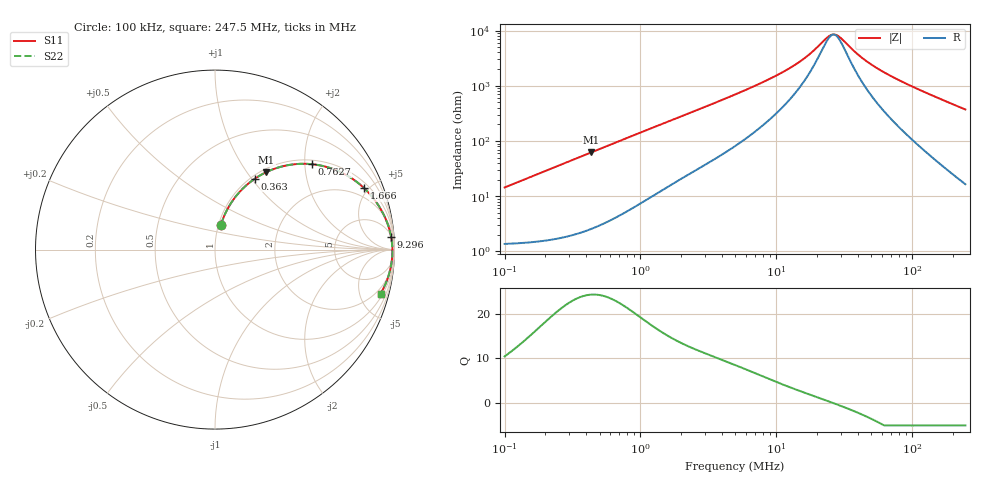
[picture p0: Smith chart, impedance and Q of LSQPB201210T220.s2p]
! LSQPB201210T220  S-PARAMETER MODEL  ( General Type )
! Model Generated by TAIYO YUDEN Corporation (http://www.ty-top.com)
! Version 2.0
! TAIYO YUDEN Control No. 100810NF18SB-HKC
! Copyright(c) 2007 TAIYO YUDEN CO.,LTD. All Rights Reserved.
! Product Description (link to TY-COMPAS)
! https://ds.yuden.co.jp/TYCOMPAS/or/detail?pn=LSQPB201210T220M&u=M
! Products Name : Inductors
! Characteristics :
!  Inductance : 22 uH , SRF(min) : 13 MHz , DC Resistance(max) : 1.69 Ohm
!  Rated Current : Saturation :190 mA , Temp Rise : 270 mA (40 degC)
!  Case Size : 2.0 x 1.25 / 0.079 x 0.049 [mm/inch] , Thickness : 1.0 / 0.04 [mm/inch]
!  (Conditions: Temperature = 25 degC , DC Bias Current/Voltage = 0A / 0V)
! External Node Assignments :
!  1  o---GGG---o  2
! GND o---------o GND
! Frequency Range : 0.1MHz  -  247.502633MHz  [ 402 STEP ]
# MHz S RI R 50
! Freq[MHz].  S11 Real  S11 Imag  S21 Real  S21 Imag  S12 Real  S12 Imag  S22 Real  S22 Imag
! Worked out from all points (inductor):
!   401 points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, 100 kHz to 247.5 MHz, reference 50 ohm
!   read as one part in series: L = 22.8 uH near 104 kHz
!   highest Q = 24.3 at 432.8 kHz (marker M1), where L = 22.7 uH
!   self-resonance near 26.44 MHz
!   S11 on the Smith chart (normalised r, x): 100 kHz: 1.03, +0.29; 363 kHz: 1.04, +1.04; 762.7 kHz: 1.10, +2.17; 1.666 MHz: 1.32, +4.67; 9.296 MHz: 6, +27; 247.5 MHz: 1.33, -7.42
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0.1  0.0328 0.1367  0.9672 -0.1367  0.9672 -0.1367  0.0328 0.1367
0.206018  0.0922 0.2636  0.9078 -0.2636  0.9078 -0.2636  0.0922 0.2636
0.363028  0.2222 0.3952  0.7778 -0.3952  0.7778 -0.3952  0.2222 0.3952
0.37019  0.2286 0.3995  0.7714 -0.3995  0.7714 -0.3995  0.2286 0.3995
0.432809  0.285 0.4313  0.715 -0.4313  0.715 -0.4313  0.285 0.4313
0.58017  0.4107 0.4713  0.5893 -0.4713  0.5893 -0.4713  0.4107 0.4713
0.76266  0.5395 0.476  0.4605 -0.476  0.4605 -0.476  0.5395 0.476
1.370406  0.7751 0.388  0.2249 -0.388  0.2249 -0.388  0.7751 0.388
1.666053  0.8293 0.3438  0.1707 -0.3438  0.1707 -0.3438  0.8293 0.3438
2.71511  0.9166 0.237  0.0834 -0.237  0.0834 -0.237  0.9166 0.237
4.974964  0.9644 0.1359  0.0356 -0.1359  0.0356 -0.1359  0.9644 0.1359
9.295576  0.9817 0.0683  0.0183 -0.0683  0.0183 -0.0683  0.9817 0.0683
13.73901  0.9859 0.0389  0.0141 -0.0389  0.0141 -0.0389  0.9859 0.0389
18.41681  0.9875 0.0206  0.0125 -0.0206  0.0125 -0.0206  0.9875 0.0206
24.20972  0.9882 0.00494  0.0118 -0.00494  0.0118 -0.00494  0.9882 0.00494
27.22034  0.9884 -0.00164  0.0116 0.00164  0.0116 0.00164  0.9884 -0.00164
30.01327  0.9884 -0.00716  0.0116 0.00716  0.0116 0.00716  0.9884 -0.00716
37.94204  0.9882 -0.0208  0.0118 0.0208  0.0118 0.0208  0.9882 -0.0208
45.23517  0.9878 -0.0318  0.0122 0.0318  0.0122 0.0318  0.9878 -0.0318
68.1772  0.985 -0.0619  0.015 0.0619  0.015 0.0619  0.985 -0.0619
122.5061  0.9732 -0.1235  0.0268 0.1235  0.0268 0.1235  0.9732 -0.1235
247.5026  0.923 -0.2453  0.077 0.2453  0.077 0.2453  0.923 -0.2453
